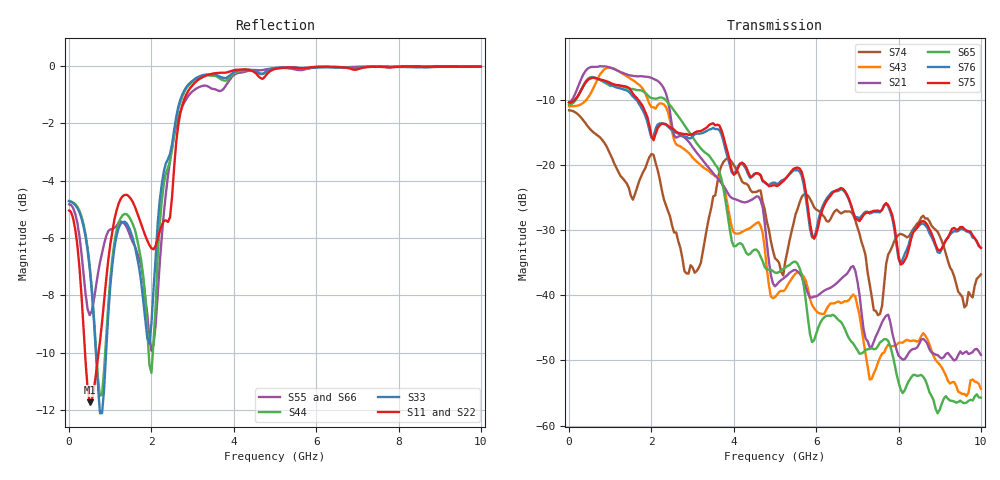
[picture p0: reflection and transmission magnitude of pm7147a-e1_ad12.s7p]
# GHz S DB R 50
! S-Parameters data
! Freq  dbS11  angS11  dbS12  angS12  dbS13  angS13  dbS14  angS14
!  dbS15  angS15  dbS16  angS16  dbS17  angS17  dbS21  angS21
!  dbS22  angS22  dbS23  angS23  dbS24  angS24  dbS25  angS25
!  dbS26  angS26  dbS27  angS27  dbS31  angS31  dbS32  angS32
!  dbS33  angS33  dbS34  angS34  dbS35  angS35  dbS36  angS36
!  dbS37  angS37  dbS41  angS41  dbS42  angS42  dbS43  angS43
!  dbS44  angS44  dbS45  angS45  dbS46  angS46  dbS47  angS47
!  dbS51  angS51  dbS52  angS52  dbS53  angS53  dbS54  angS54
!  dbS55  angS55  dbS56  angS56  dbS57  angS57  dbS61  angS61
!  dbS62  angS62  dbS63  angS63  dbS64  angS64  dbS65  angS65
!  dbS66  angS66  dbS67  angS67  dbS71  angS71  dbS72  angS72
!  dbS73  angS73  dbS74  angS74  dbS75  angS75  dbS76  angS76
!  dbS77  angS77
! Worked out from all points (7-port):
!   279 points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, 1 Hz to 10 GHz, reference 50 ohm
!   strongest paths, dB at 1 Hz, 7.943 MHz, 3.05 GHz, 6.55 GHz, 10 GHz:
!     S75: -10.4, -10.4, -15.0, -23.7, -32.7
!     S76: -10.4, -10.4, -15.3, -23.9, -32.7
!     S65: -10.7, -10.7, -16.2, -43.8, -55.7
!     S21: -10.3, -10.3, -17.7, -37.8, -49.1
!     S43: -11.0, -11.0, -19.2, -41.0, -54.3
!     S74: -11.6, -11.6, -36.5, -27.2, -36.8
!   lowest |S11| = -11.7 dB at 500 MHz (marker M1), VSWR 1.70, Z = 29.4 + j1.21 ohm
!   |S11| at or under -10 dB: 387.1 MHz to 714.7 MHz (327.6 MHz wide, 59.5 % of centre)
